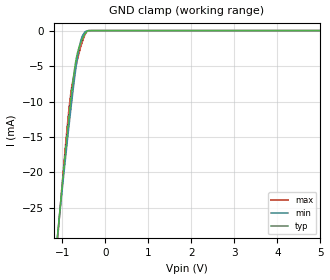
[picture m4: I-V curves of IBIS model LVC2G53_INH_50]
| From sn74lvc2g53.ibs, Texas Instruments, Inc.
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[Model]   LVC2G53_INH_50
Model_type  Input
Vinl=1.35
Vinh=3.85
| variable   typ   min   max
C_comp   3.73pF   2.65pF   6.34pF
[Temperature Range]   40   100   -40
| Ambient temperature   25   85   -40
[Voltage range]   5   4.5   5.5
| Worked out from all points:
|   GND clamp passes 1 mA (typ) near -0.52 V on its own axis
[GND Clamp]
| LVC2G53_INH_50
|   Voltage   I(typ)   I(min)   I(max)
-5.5V     -348.1mA   -320.8mA   -389.9mA
-1.095V   -28.11mA   -28.23mA   -28.63mA
-1.055V   -25.49mA   -25.83mA   -25.68mA
-885mV    -14.76mA   -15.92mA   -13.77mA
-830mV    -11.51mA   -12.86mA   -10.43mA
-790mV    -9.266mA   -10.72mA   -8.474mA
-695mV    -4.747mA   -5.983mA   -5.424mA
-655mV    -3.439mA   -4.243mA   -4.362mA
-605mV    -2.342mA   -2.43mA    -3.134mA
-530mV    -1.194mA   -768.4uA   -1.547mA
-435mV    -182.9uA   -61.02uA   -202.3uA
5V        210.6pA    655.8pA    1.541nA
